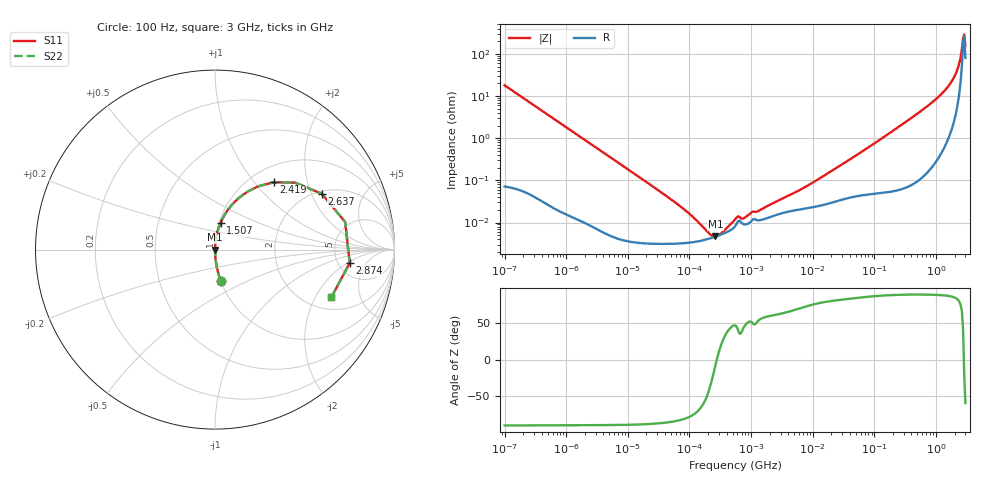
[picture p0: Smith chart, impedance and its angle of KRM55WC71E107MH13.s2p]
!Murata Part Number: KRM55WC71E107MH13
!These Parameters are Measured in Series Mode Connection
!Data Generated on Jan 08, 2026
!  o--ll--o
!Port1  Port2
!  o------o
!Operation Temp=25[degC], DC Bias Voltage=0[V]
!Freq. Start=100[Hz] Stop=3[GHz] 401[Steps]
# Hz S RI R 50
!Freq.(Hz) S11(Real) S11(Imag) S21(Real) S21(Imag) S12(Real) S12(Imag) S22(Real) S22(Imag)
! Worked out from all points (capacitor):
!   401 points, 100 Hz to 3 GHz, reference 50 ohm
!   read as one part in series: C = 88.5 uF near 109 Hz
!   lowest |Z| = 4.66 mohm at 263.5 kHz (marker M1)
!   series resonance near 277.7 kHz, so ESL is about 3.7 nH
!   S11 on the Smith chart (normalised r, x): 100 Hz: 1.00, -0.36; 1.507 GHz: 1.02, +0.31; 2.419 GHz: 1.27, +1.26; 2.637 GHz: 2.11, +2.39; 2.874 GHz: 6.35, -2.20; 3 GHz: 2.61, -2.73
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100  0.032 -0.174  0.968 0.174  0.968 0.174  0.032 -0.174
306  0.00387 -0.0587  0.9961 0.0587  0.9961 0.0587  0.00387 -0.0587
1788  0.000209 -0.0102  0.9998 0.0102  0.9998 0.0102  0.000209 -0.0102
31977  3.14e-05 -0.000565  1 0.000565  1 0.000565  3.14e-05 -0.000565
138163  3.57e-05 -9.68e-05  1 9.68e-05  1 9.68e-05  3.57e-05 -9.68e-05
263501  4.62e-05 -6.3e-06  1 6.3e-06  1 6.3e-06  4.62e-05 -6.3e-06
461094  6.54e-05 6.11e-05  0.9999 -6.11e-05  0.9999 -6.11e-05  6.54e-05 6.11e-05
547723  8.11e-05 8.57e-05  0.9999 -8.57e-05  0.9999 -8.57e-05  8.11e-05 8.57e-05
623217  0.000109 8.72e-05  0.9999 -8.72e-05  0.9999 -8.72e-05  0.000109 8.72e-05
772864  9.04e-05 9.01e-05  0.9999 -9.01e-05  0.9999 -9.01e-05  9.04e-05 9.01e-05
1000599  0.000106 0.000134  0.9999 -0.000134  0.9999 -0.000134  0.000106 0.000134
1352413  0.000113 0.000155  0.9999 -0.000155  0.9999 -0.000155  0.000113 0.000155
9794414  0.00023 0.000837  0.9998 -0.000837  0.9998 -0.000837  0.00023 0.000837
1.751444e8  0.000701 0.0131  0.9993 -0.0131  0.9993 -0.0131  0.000701 0.0131
7.567485e8  0.00527 0.0601  0.9947 -0.0601  0.9947 -0.0601  0.00527 0.0601
1.506733e9  0.0312 0.1494  0.9688 -0.1494  0.9688 -0.1494  0.0312 0.1494
2.036508e9  0.1102 0.2667  0.8898 -0.2667  0.8898 -0.2667  0.1102 0.2667
2.219584e9  0.1817 0.3233  0.8183 -0.3233  0.8183 -0.3233  0.1817 0.3233
2.419119e9  0.3269 0.3752  0.6731 -0.3752  0.6731 -0.3752  0.3269 0.3752
2.636591e9  0.5952 0.3112  0.4048 -0.3112  0.4048 -0.3112  0.5952 0.3112
2.873614e9  0.7503 -0.0747  0.2497 0.0747  0.2497 0.0747  0.7503 -0.0747
3e9  0.6481 -0.2663  0.3519 0.2663  0.3519 0.2663  0.6481 -0.2663
